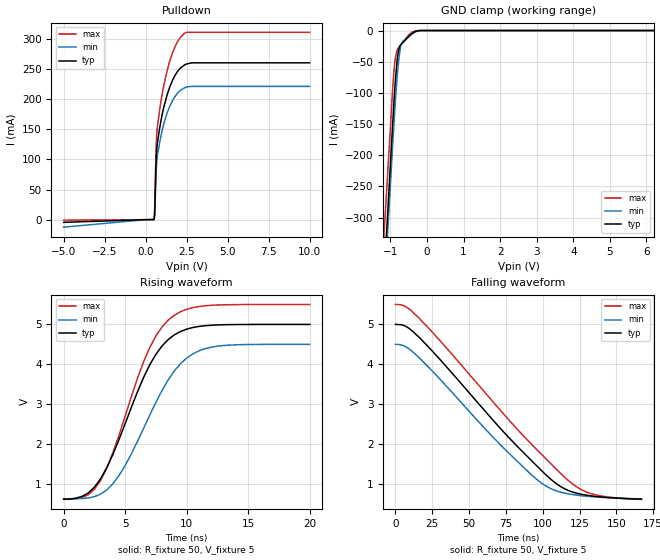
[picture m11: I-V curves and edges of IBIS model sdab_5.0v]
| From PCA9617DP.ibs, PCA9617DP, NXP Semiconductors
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[Model]   sdab_5.0v
Model_type Open_drain
Vref=5.000E+00
Rref=1.350E+03
Cref=5.000E-11
Vmeas=2.500E+00
C_comp   8.050E-13   7.840E-13   8.260E-13
[Voltage Range]   5.000E+00   4.500E+00   5.500E+00
[POWER Clamp Reference]   5.000E+00   4.500E+00   5.500E+00
[GND Clamp Reference]   0.000E+00   0.000E+00   0.000E+00
[Pullup Reference]   5.000E+00   4.500E+00   5.500E+00
[Pulldown Reference]   0.000E+00   0.000E+00   0.000E+00
[Temperature Range]   25   85   -40
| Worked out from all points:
|   slope of the pulldown table from 0 to 0.75 V, typ, clamps not added: 5.59 ohm
|   GND clamp passes 1 mA (typ) near -0.29 V on its own axis
|   rising waveform, R_fixture 50, V_fixture 5: 20-80 % time 3.62ns typ, 3.88ns min, 3.42ns max; typ from 0.615 V to 5 V
|   falling waveform, R_fixture 50, V_fixture 5: 20-80 % time 64.6ns typ, 59.7ns min, 71.3ns max; typ from 5 V to 0.615 V
[GND Clamp]
-5V       -4.401A    -4.288A    -4.055A
-1V       -212.4mA   -244.7mA   -153.8mA
-940mV    -149.1mA   -184mA     -93.24mA
-880mV    -91.39mA   -125.7mA   -49.77mA
-820mV    -48.76mA   -76.05mA   -32.03mA
-800mV    -39.12mA   -62.36mA   -29.51mA
-740mV    -24.69mA   -32.18mA   -24.85mA
-700mV    -21.42mA   -21.32mA   -21.87mA
-660mV    -19.24mA   -16.96mA   -18.7mA
-460mV    -7.047mA   -7.953mA   -4.982mA
-320mV    -1.603mA   -2.28mA    -684.3uA
10V       0A         0A         0A
[Pulldown]
-5V       -4.402mA   -12.44mA   -771.8uA
500mV     97.73uA    97.97uA    335.2uA
540mV     7.04mA     4.979mA    11.48mA
560mV     20.66mA    15.34mA    29.34mA
620mV     84.74mA    68.25mA    105.4mA
660mV     110.6mA    90.61mA    135.1mA
740mV     132.4mA    110.2mA    159.8mA
980mV     171.3mA    145.4mA    204.7mA
1.3V      206.5mA    176.4mA    246.6mA
1.64V     231.6mA    197.9mA    277.4mA
2.36V     256.8mA    218.9mA    309.3mA
10V       260.5mA    221.3mA    311.1mA
[Rising Waveform]
R_fixture = 50
V_fixture = 5
V_fixture_min = 4.5
V_fixture_max = 5.5
0s        615.1mV    621.1mV    608.5mV
2ns       769.3mV    643.7mV    724.3mV
3ns       1.126V     739mV      1.084V
4.5ns     2.112V     1.206V     2.224V
7ns       3.988V     2.725V     4.422V
8ns       4.461V     3.344V     4.939V
9ns       4.738V     3.833V     5.232V
10.5ns    4.922V     4.262V     5.421V
12ns      4.979V     4.428V     5.479V
20ns      5V         4.5V       5.5V
[Falling Waveform]
R_fixture = 50
V_fixture = 5
V_fixture_min = 4.5
V_fixture_max = 5.5
0s        5V         4.5V       5.5V
7ns       4.952V     4.438V     5.445V
16.5ns    4.66V      4.148V     5.14V
71ns      2.399V     1.986V     2.854V
92.5ns    1.575V     1.218V     1.984V
101.5ns   1.246V     957.3mV    1.651V
114.5ns   880.1mV    767.1mV    1.175V
129.5ns   713.3mV    687.4mV    794.8mV
144ns     654.3mV    649.6mV    668.7mV
167ns     615.1mV    621.1mV    608.5mV
[Ramp]
dV/dt_r   2.6310E+00/3.6030E-09   2.3273E+00/3.8620E-09   2.9349E+00/3.3960E-09
dV/dt_f   2.6310E+00/6.4634E-08   2.3273E+00/5.9602E-08   2.9349E+00/7.1344E-08
R_load = 50
